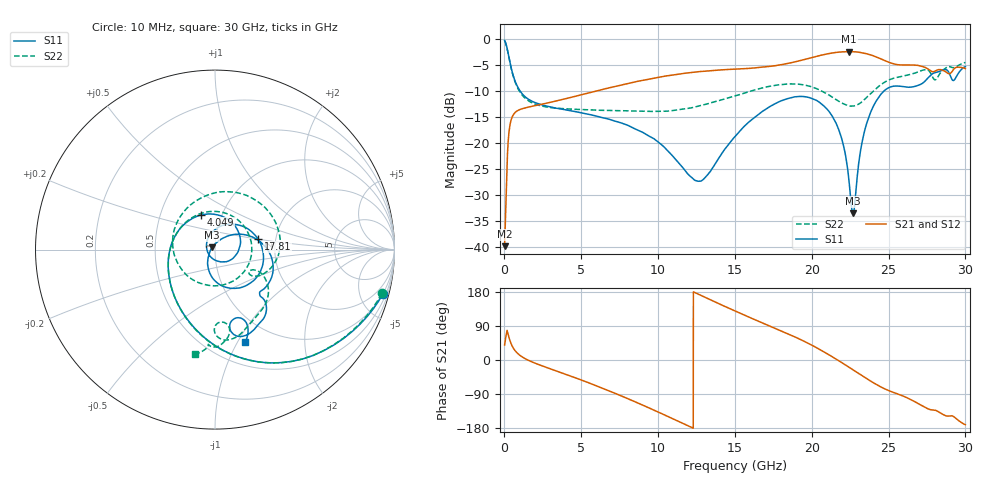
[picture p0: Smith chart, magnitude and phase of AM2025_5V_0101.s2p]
!Keysight Technologies,N5245B,MY58422270,A.16.20.02
!Date: Tuesday, July 14, 2026 01:04:13
!Correction: S11(C  2-Port  )
!S21(C  2-Port  )
!S12(C  2-Port  )
!S22(C  2-Port  )
!S2P File: Measurements: S11, S21, S12, S22:
# Hz S  dB  R 50
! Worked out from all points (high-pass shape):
!   3201 points, 10 MHz to 30 GHz, reference 50 ohm
!   highest |S21| = -2.43 dB at 22.43 GHz (marker M1); lowest = -39.8 dB at 10 MHz (marker M2)
!   |S21| within 3 dB of the highest: 16.76 GHz to 27.34 GHz (10.59 GHz wide, 48 % of centre); 29.46939 GHz to 29.59898 GHz (129.6 MHz wide, 0.439 % of centre)
!   lowest |S11| = -33.5 dB at 22.69 GHz (marker M3), VSWR 1.04, Z = 48.3 + j1.2 ohm
!   |S11| at or under -10 dB: 1.018 GHz to 24.7 GHz (23.68 GHz wide, 184 % of centre)
!   |S22| runs from -13.9 to -0.3 dB; largest |S21 - S12| = 0.0065
!   S11 on the Smith chart (normalised r, x): 10 MHz: 1.00, -7.52; 4.049 GHz: 0.80, +0.32; 17.81 GHz: 1.61, +0.20; 30 GHz: 0.74, -1.08
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1e7  -0.30 -14.9  -39.78 39.6  -39.15 69.5  -0.35 -14.7
3.286438e8  -4.09 -75.8  -17.11 54.8  -17.11 54.9  -4.14 -76.5
5.34825e8  -6.69 -102.4  -14.78 34.2  -14.78 34.1  -6.77 -103.7
8.253531e8  -9.01 -128.0  -13.82 18.6  -13.82 18.5  -9.21 -130.5
2.099928e9  -12.34 169.3  -12.74 -10.1  -12.73 -10.1  -12.64 159.8
4.049278e9  -13.65 112.2  -11.42 -38.7  -11.42 -38.7  -13.43 92.3
5.014581e9  -14.20 88.2  -10.71 -53.0  -10.70 -53.1  -13.56 63.4
7.460641e9  -16.00 29.7  -8.93 -92.3  -8.93 -92.3  -13.76 -8.2
1.000979e10  -19.80 -35.8  -7.37 -137.4  -7.37 -137.4  -13.91 -86.5
1.269015e10  -27.32 -159.1  -6.27 172.4  -6.27 172.3  -12.84 -171.6
1.5005e10  -18.74 87.5  -5.79 129.3  -5.79 129.2  -10.93 118.7
1.780719e10  -12.16 13.9  -5.05 80.4  -5.04 80.4  -8.83 43.3
2.000958e10  -11.44 -46.5  -3.57 39.0  -3.57 39.0  -9.21 -9.8
2.161217e10  -16.36 -97.2  -2.59 1.7  -2.59 1.7  -11.70 -34.7
2.242752e10  -27.31 -140.7  -2.43 -19.1  -2.44 -19.2  -12.84 -34.2
2.268994e10  -33.46 144.2  -2.46 -26.0  -2.46 -26.1  -12.90 -31.9
2.356152e10  -16.33 34.4  -2.84 -48.9  -2.84 -48.9  -11.26 -26.6
2.500479e10  -9.37 -17.6  -4.47 -80.7  -4.47 -80.7  -7.90 -43.9
2.73665e10  -8.12 -45.7  -5.46 -124.7  -5.45 -124.8  -5.90 -79.5
2.806002e10  -6.45 -57.4  -6.13 -132.9  -6.12 -132.9  -7.83 -84.1
2.901595e10  -7.08 -79.3  -6.63 -147.3  -6.61 -147.5  -5.36 -92.5
3e10  -5.32 -72.0  -5.69 -170.6  -5.65 -171.1  -4.53 -100.9
